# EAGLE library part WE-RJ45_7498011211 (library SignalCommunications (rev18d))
Order Code 7498011211 Design SMD xBase-T 10/100 Base-T Ports 1x1 Application Standard Tab Position DOWN LED (Left-Right) GREEN-YELLOW EMI Fingers Yes Details see: http://katalog.we-online.de/en/pbs/WE-LAN_RJ45/7498011211? Updated by Yingchun Shan 2016-08-23 2014 (C) Würth Elektronik
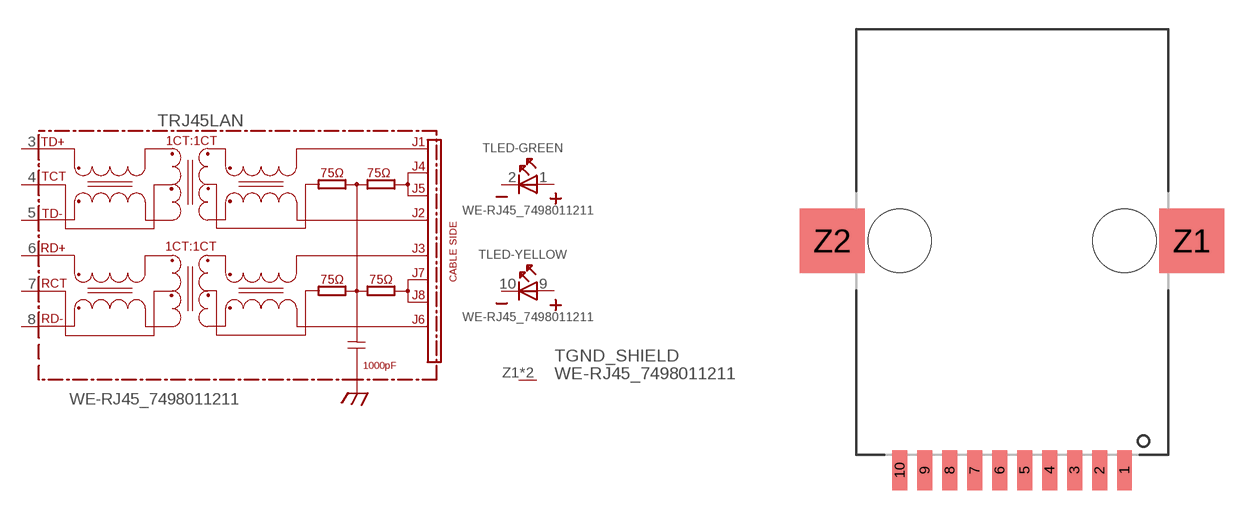
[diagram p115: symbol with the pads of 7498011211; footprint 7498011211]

Designator prefix T; gates RJ45LAN=7498011211 LED-GREEN=LED2PIN LED-YELLOW=LED2PIN GND_SHIELD=GNDPIN

## WE-RJ45_7498011211 (COMPANY-URL: http://www.we-online.de; CREATED-BY: Christin Zierenner; CREATED-DATE: AUG 2012; DATASHEET-URL: http://katalog.we-online.de/kataloge/eisos/media/pdf/7498011211.pdf; MANUFACTURER: Würth Elektronik eiSos GmbH)  [7498011211]
1  LED-GREEN:A  pas
2  LED-GREEN:K  pas
3  RJ45LAN:TD+
4  RJ45LAN:TCT
5  RJ45LAN:TD-
6  RJ45LAN:RD+
7  RJ45LAN:RCT
8  RJ45LAN:RD-
9  LED-YELLOW:A  pas
10  LED-YELLOW:K  pas
Z1  GND_SHIELD:GND  pwr
Z2  GND_SHIELD:GND  pwr

## Footprint 7498011211 (pad centres in mm)
MAX HEIGHT=13.50mm PORTS----1X1 LED --Yes
smd 0.76 x 2.03: 1 5.715,-11.68; 2 4.445,-11.68; 3 3.175,-11.68; 4 1.905,-11.68; 5 0.635,-11.68; 6 -0.635,-11.68; 7 -1.905,-11.68; 8 -3.175,-11.68; 9 -4.445,-11.68; 10 -5.715,-11.68
smd 3.3 x 3.3: Z1 9.145,0; Z2 -9.145,0
hole 3.22 at -5.715,0
hole 3.22 at 5.715,0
